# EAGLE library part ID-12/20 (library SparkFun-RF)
ID Innovations 125kHz RFID Reader (ID2, ID3, ID12, and ID20) The IDS, ID3, ID12, and ID20 are very simple to use RFID reader modules. Power the module, hold up a 125kHz card, and get a serial string output containing the unique ID of the card. SparkFun Products RFID Reader ID-3LA (125 kHz) (SEN-11862) RFID Reader ID-12LA (125 kHz) (SEN-11827) RFID Reader ID-20LA (125 kHz) (SEN-11828) SparkFun RFID USB Reader (SEN-9963)
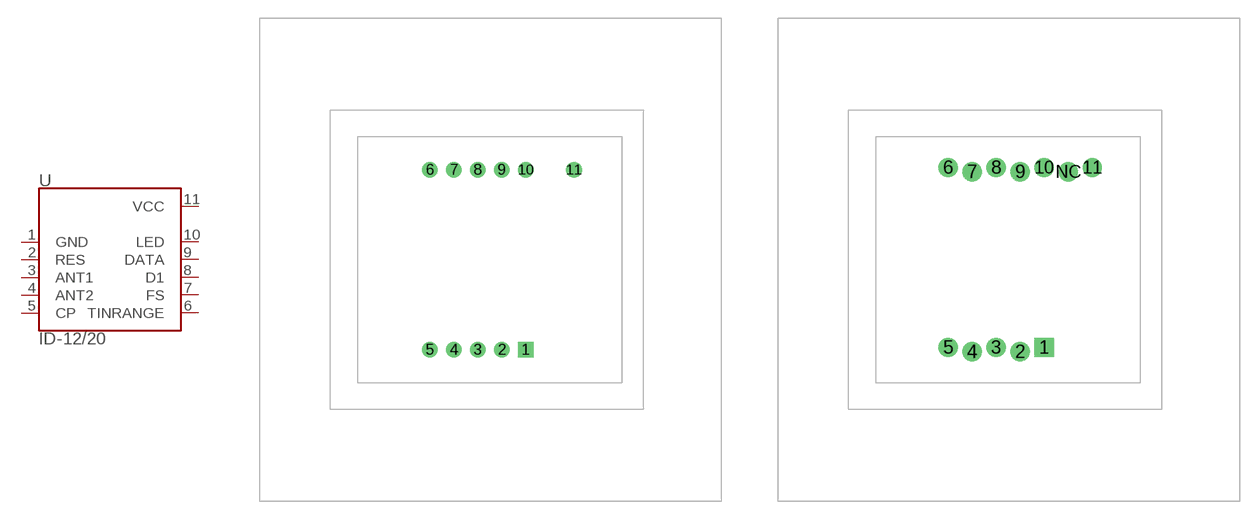
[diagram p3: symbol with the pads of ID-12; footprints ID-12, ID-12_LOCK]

Designator prefix U

## ID-12/20 (PROD_ID: CONN-08875)  [ID-12]
1  GND
2  RES
3  ANT1
4  ANT2
5  CP
6  TINRANGE
7  FS
8  D1
9  DATA
10  LED
11  VCC

## ID-12/20ID-12_LOCK (PROD_ID: CONN-08875)  [ID-12_LOCK]
Pads as for ID-12

## ID-12/20SMD (PROD_ID: CONN-09345, CONN-09344)  [ID-12_SMD]
Pads as for ID-12

## Footprint ID-12 (pad centres in mm)
ID-2, ID-12, and ID-20 Low-voltage RFID Readers Footprint works for ID-2LA, ID-12LA, and ID-20LA modules Dimensions of RFID readers vary, but the pin-out remains the same. Datasheet
drill 0.8 square: 1 3,-7.5
drill 0.8: 2 1,-7.5; 3 -1,-7.5; 4 -3,-7.5; 5 -5,-7.5; 6 -5,7.5; 7 -3,7.5; 8 -1,7.5; 9 1,7.5; 10 3,7.5; 11 7,7.5

## Footprint ID-12_LOCK (pad centres in mm)
ID-2, ID-12, and ID-20 Low-voltage RFID Readers Locking PTH footprint! Adjacent holes are offset. Footprint works for ID-2LA, ID-12LA, and ID-20LA modules Dimensions of RFID readers vary, but the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
drill 0.737 pad 1.6 square: 1 2.999,-7.311
drill 0.737 pad 1.6: 2 0.999,-7.666; 3 -1.001,-7.311; 4 -3.001,-7.666; 5 -5.001,-7.311; 6 -5.001,7.689; 7 -3.001,7.334; 8 -1.001,7.689; 9 0.999,7.334; 10 2.999,7.689; 11 6.999,7.689; NC 5.012,7.334

## Footprint ID-12_SMD (pad centres in mm)
ID-2, ID-12, and ID-20 Low-voltage RFID Readers - SMD Footprint Footprint works for ID-2LA, ID-12LA, and ID-20LA modules Dimensions of RFID readers vary, but the pin-out remains the same. Datasheet
smd 0.85 x 1.7: 1 2.993,-8.998; 2 0.993,-5.998; 3 -1.007,-8.998; 4 -3.007,-5.998; 5 -5.007,-8.998; 6 -5.007,6.013; 7 -3.007,9.013; 8 -1.007,6.013; 9 0.993,9.013; 10 2.993,6.013; 11 6.993,6.013; NC 4.993,9.013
